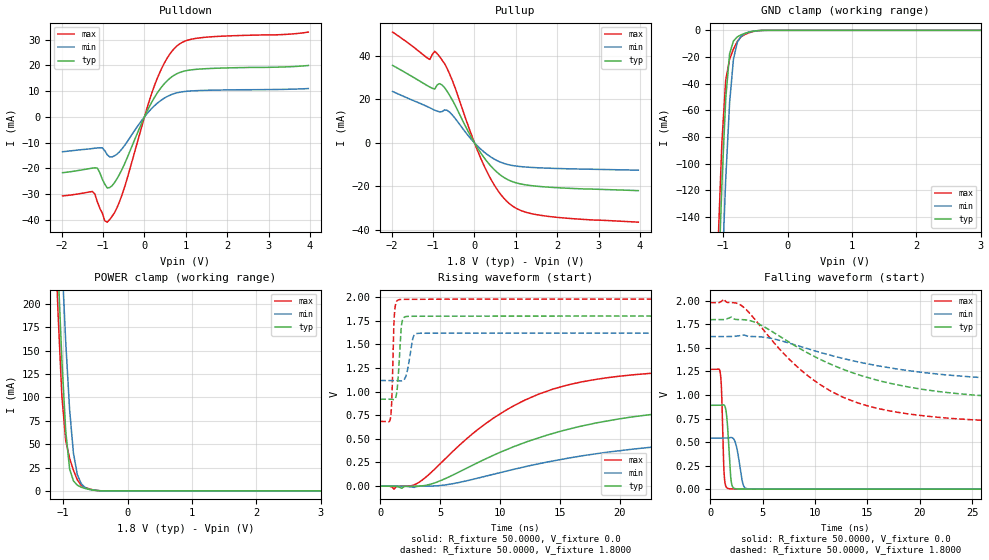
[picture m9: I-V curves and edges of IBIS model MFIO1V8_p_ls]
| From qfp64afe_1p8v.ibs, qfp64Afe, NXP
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[Model] MFIO1V8_p_ls
|   Model MFIO1V8_p_ls
| This model was characterised for following simulation conditions:
| External (pad) voltage:
|   - Typ: 1.8V,   - Min: 1.62V,   - Max: 1.98V
| Library cells for typ/min/max conditions are connected as defined below:
|  IO - External Pad
|  A - Core Input
|  EN - Output Buffer Enable
|  BOOST - vdde
|  EHS - gnd
|  ENZI - vdd
|  EPD - gnd
|  EPUN - vdd
|  ZI - NC
|  ZIF - NC
|  gnd - gnd
|  gnde - gnde
|  vdd - vdd
|  vdde - vdde
| All other pins connected to ground
Model_type I/O
Polarity   Non-Inverting
Enable   Active-Low
Vinl =   0.5400V
Vinh =   1.2600V
Vmeas =  0.9000V
Cref =   0.0F
Rref =   100.0000
Vref =   0.0V
C_comp   1.6238pF   1.5412pF   1.6971pF
|C_comp_pullup   0.8047pF   0.8356pF   0.7616pF
|C_comp_pulldown   0.6044pF   0.6428pF   0.5687pF
[Model Spec]
| variable   typ   min   max
Vinh   0.5400V   0.4860V   0.5940V
Vinl   1.2600V   1.1340V   1.3860V
Vmeas   0.9000V   0.8100V   0.9900V
[Temperature Range]   25.0000   0.1250k   -40.0000
[Voltage Range]   1.8000V   1.6200V   1.9800V
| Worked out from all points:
|   slope of the pulldown table from 0 to 0.27 V, typ, clamps not added: 32.6 ohm
|   slope of the pullup table from 0 to 0.27 V, typ, clamps not added: 34.8 ohm
|   GND clamp passes 1 mA (typ) near -0.56 V on its own axis
|   POWER clamp passes 1 mA (typ) near -0.54 V on its own axis
|   rising waveform, R_fixture 50.0000, V_fixture 0.0: 20-80 % time 13ns typ, 15.7ns min, 9.08ns max; typ from 0 V to 0.89 V
|   rising waveform, R_fixture 50.0000, V_fixture 1.8000: 20-80 % time 250ps typ, 394ps min, 169ps max; typ from 0.92 V to 1.8 V
|   falling waveform, R_fixture 50.0000, V_fixture 0.0: 20-80 % time 296ps typ, 476ps min, 197ps max; typ from 0.89 V to 0 V
|   falling waveform, R_fixture 50.0000, V_fixture 1.8000: 20-80 % time 11.8ns typ, 13.6ns min, 8.55ns max; typ from 1.8 V to 0.92 V
[Pulldown]
|Voltage   I(typ)   I(min)   I(max)
-1.98V    -21.74mA   -13.58mA   -30.76mA
-1.26V    -19.96mA   -12.33mA   -29.04mA
-1.14V    -19.96mA   -12.1mA    -33mA
-960mV    -26.19mA   -13.15mA   -40.44mA
-840mV    -27.51mA   -15.58mA   -39.92mA
-540mV    -20.34mA   -12.41mA   -30.2mA
60mV      2.086mA    1.197mA    3.341mA
300mV     9.043mA    5.145mA    14.58mA
540mV     13.88mA    7.813mA    22.59mA
840mV     17.16mA    9.517mA    28.23mA
1.44V     18.67mA    10.27mA    30.87mA
3.96V     19.95mA    10.98mA    32.93mA
[Pullup]
|Voltage   I(typ)   I(min)   I(max)
-1.98V    35.7mA     23.68mA    51.03mA
-1.08V    25.71mA    16.17mA    38.42mA
-960mV    24.81mA    15.04mA    42.18mA
-840mV    27.29mA    14.27mA    39.65mA
-720mV    25.36mA    15.21mA    36.42mA
-540mV    19.88mA    12.94mA    28.95mA
-60mV     2.002mA    1.263mA    3.041mA
240mV     -7.02mA    -4.333mA   -10.88mA
600mV     -14.41mA   -8.644mA   -22.88mA
900mV     -17.74mA   -10.36mA   -28.83mA
1.74V     -20.33mA   -11.62mA   -33.75mA
3.96V     -22mA      -12.58mA   -36.53mA
[GND_clamp]
|Voltage   I(typ)   I(min)   I(max)
-1.98V    -1.781A    -1.801A    -1.77A
-1.08V    -200.1mA   -270.2mA   -162.2mA
-1.02V    -116mA     -186.2mA   -84.48mA
-960mV    -51.25mA   -111.8mA   -37.35mA
-900mV    -17.64mA   -54.43mA   -21.68mA
-840mV    -8.011mA   -21.69mA   -14.07mA
-780mV    -4.915mA   -8.957mA   -8.303mA
-720mV    -3.329mA   -4.435mA   -4.743mA
-600mV    -1.395mA   -1.331mA   -1.886mA
-480mV    -322.5uA   -340.7uA   -414uA
-360mV    -20uA      -33.74uA   -21.95uA
3.96V     0A         0A         0A
[POWER_clamp]
|Voltage   I(typ)   I(min)   I(max)
-1.98V    2.119A     2.147A     2.105A
-1.14V    349.2mA    449.9mA    300.5mA
-1.08V    239.1mA    345.9mA    191.2mA
-1.02V    140.3mA    247.7mA    101.6mA
-960mV    64.04mA    159.3mA    53.83mA
-900mV    23.55mA    87.2mA     35.06mA
-840mV    10.74mA    40.16mA    22.02mA
-780mV    6.173mA    17.47mA    11.87mA
-720mV    3.968mA    7.718mA    5.953mA
-600mV    1.695mA    1.811mA    2.312mA
-360mV    25.02uA    62.74uA    19.06uA
3.96V     0A         0A         0A
[Ramp]
| variable   typ   min   max
dV/dt_r  0.5342/12.9695n   0.3253/15.7103n   0.7634/9.0766n
dV/dt_f  0.5278/11.7673n   0.3012/13.6098n   0.7772/8.5555n
R_load = 50.0000
[Rising Waveform]
R_fixture= 50.0000
V_fixture= 0.0
V_fixture_min= 0.0
V_fixture_max= 0.0
|time   V(typ)   V(min)   V(max)
0s        1.152nV    106.1nV    55.38pV
1.154ns   -116uV     27.77uV    -32.39mV
3.182ns   -284.7uV   -2.126mV   35.62mV
4.939ns   52.5mV     5.255mV    228.5mV
8.619ns   277.5mV    98.99mV    644.9mV
12.1ns    462.6mV    205.2mV    911.6mV
15.71ns   601.7mV    296.1mV    1.072V
20.97ns   731mV      389.8mV    1.177V
40.29ns   869mV      517.1mV    1.262V
100ns     890.3mV    542.2mV    1.272V
[Rising Waveform]
R_fixture= 50.0000
V_fixture= 1.8000
V_fixture_min= 1.6200
V_fixture_max= 1.9800
|time   V(typ)   V(min)   V(max)
0s        920.2mV    1.118V     684.7mV
847.2ps   920.4mV    1.118V     716.9mV
968.2ps   918.5mV    1.118V     928.6mV
1.202ns   917.5mV    1.118V     1.853V
1.44ns    1.062V     1.117V     1.966V
1.672ns   1.54V      1.114V     1.976V
1.95ns    1.782V     1.121V     1.977V
2.738ns   1.798V     1.571V     1.978V
3.277ns   1.798V     1.618V     1.978V
100ns     1.8V       1.62V      1.98V
[Falling Waveform]
R_fixture= 50.0000
V_fixture= 0.0
V_fixture_min= 0.0
V_fixture_max= 0.0
|time   V(typ)   V(min)   V(max)
0s        890.4mV    542.3mV    1.272V
953.6ps   890.6mV    542.4mV    1.237V
1.079ns   892.5mV    542.3mV    1.043V
1.346ns   890.8mV    542.2mV    127.1mV
1.579ns   763.4mV    543.2mV    14.81mV
1.808ns   376.7mV    546.2mV    4.071mV
2.13ns    26.31mV    544.4mV    2.08mV
3.154ns   1.326mV    42.47mV    1.743mV
3.778ns   1.333mV    1.86mV     1.27mV
100ns     20.58nV    164nV      7.285nV
[Falling Waveform]
R_fixture= 50.0000
V_fixture= 1.8000
V_fixture_min= 1.6200
V_fixture_max= 1.9800
|time   V(typ)   V(min)   V(max)
0s        1.8V       1.62V      1.98V
1.307ns   1.801V     1.62V      2.019V
3.054ns   1.8V       1.635V     1.944V
4.713ns   1.75V      1.618V     1.741V
7.825ns   1.541V     1.542V     1.349V
11.52ns   1.326V     1.421V     1.04V
15.01ns   1.186V     1.331V     884.6mV
20.3ns    1.06V      1.24V      779.5mV
40.29ns   936.1mV    1.132V     693.5mV
100ns     920.3mV    1.118V     684.7mV
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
